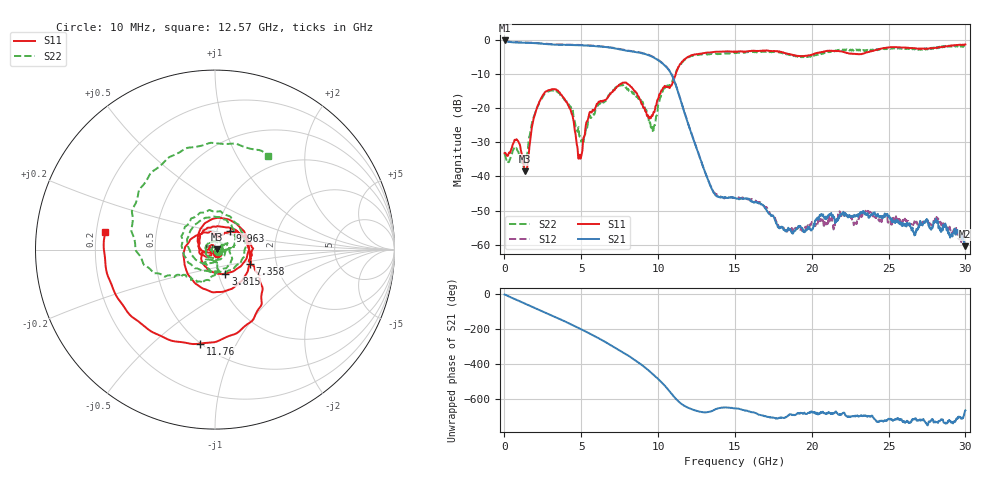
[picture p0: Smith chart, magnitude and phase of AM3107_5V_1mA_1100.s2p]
# Hz S DB R 50.0
!freq dBS11 angS11 dBS21 angS21 dBS12 angS12 dBS22 angS22
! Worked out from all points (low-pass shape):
!   1601 points, 10 MHz to 30 GHz, reference 50 ohm
!   highest |S21| = -0.12 dB at 10 MHz (marker M1); lowest = -60.4 dB at 29.96 GHz (marker M2)
!   |S21| within 3 dB of the highest: start of sweep to 7.937 GHz
!   lowest |S11| = -38.5 dB at 1.36 GHz (marker M3), VSWR 1.02, Z = 51.2 + j0.279 ohm
!   |S11| at or under -10 dB: start of sweep to 11.15 GHz
!   |S22| runs from -37.2 to -1.6 dB; largest |S21 - S12| = 0.012
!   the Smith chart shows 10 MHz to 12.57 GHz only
!   S11 on the Smith chart (normalised r, x): 10 MHz: 1.02, -0.04; 3.815 GHz: 1.08, -0.30; 7.358 GHz: 1.46, -0.24; 9.963 GHz: 1.16, +0.24; 11.76 GHz: 0.50, -0.72; 12.57 GHz: 0.24, +0.08
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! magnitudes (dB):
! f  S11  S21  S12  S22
! 10 MHz  -33.1  -0.1  -0.1  -33.3
! 816 MHz  -29.2  -0.7  -0.6  -32.2
! 1.36 GHz  -38.5  -0.8  -0.7  -35.1
! 2.39 GHz  -17.0  -1.0  -1.0  -17.3
! 3.815 GHz  -16.7  -1.4  -1.3  -16.9
! 5.015 GHz  -33.5  -1.6  -1.5  -29.7
! 5.614 GHz  -21.1  -1.7  -1.6  -22.8
! 7.358 GHz  -13.6  -2.6  -2.5  -13.6
! 8.97 GHz  -18.8  -3.9  -3.8  -18.2
! 9.569 GHz  -22.2  -4.8  -4.7  -26.2
! 9.963 GHz  -17.5  -5.8  -5.7  -20.9
! 10.02 GHz  -17.1  -6.0  -5.8  -18.9
! 10.88 GHz  -13.3  -10.2  -10.1  -12.4
! 11.76 GHz  -5.5  -21.9  -21.9  -5.7
! 12.57 GHz  -4.2  -32.5  -32.5  -4.4
! 13.69 GHz  -3.5  -45.2  -44.9  -4.0
! 15.01 GHz  -3.3  -46.3  -46.3  -3.8
! 18.36 GHz  -3.9  -55.9  -56.1  -4.2
! 20.01 GHz  -4.3  -55.6  -53.3  -4.7
! 25.01 GHz  -2.2  -51.7  -53.4  -2.6
! 29.96 GHz  -1.3  -60.4  -56.9  -1.8
! 30 GHz  -1.3  -60.0  -56.7  -1.6
